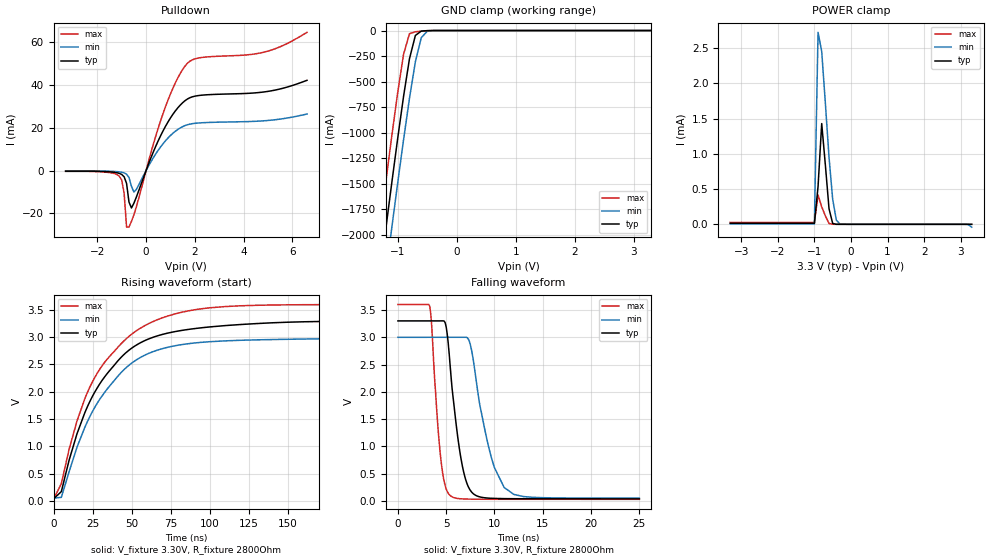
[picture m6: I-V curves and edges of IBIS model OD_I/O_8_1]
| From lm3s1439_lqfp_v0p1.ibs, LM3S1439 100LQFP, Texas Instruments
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[Model]   OD_I/O_8_1
Model_type   I/O_open_drain
Polarity   Inverting
Vinl = 1.26
Vinh = 2.04
Vmeas = 1.65
Rref = 2800
Vref = 3.3
| variable   typ   min   max
C_comp   9.739pF   9.739pF   9.739pF
[Model Spec]
Vinh+   1.91   1.78   2.04
Vinh-   1.90   1.76   2.03
Vinl+   1.40   1.27   1.54
Vinl-   1.39   1.26   1.53
| variable   typ   min   max
[Temperature Range]  25   85   -40
[Voltage Range]   3.3V   3.0V   3.6V
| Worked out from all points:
|   slope of the pulldown table from 0 to 0.495 V, typ, clamps not added: 35.8 ohm
|   GND clamp passes 1 mA (typ) near -0.48 V on its own axis
|   POWER clamp passes 1 mA (typ) near -0.73 V on its own axis
|   falling waveform, V_fixture 3.30V, R_fixture 2800Ohm: 20-80 % time 1.29ns typ, 1.99ns min, 858ps max; typ from 3.3 V to 0.038 V
|   rising waveform, V_fixture 3.30V, R_fixture 2800Ohm: 20-80 % time 34.3ns typ, 34ns min, 35.1ns max; typ from 0.038 V to 3.3 V
[Pulldown]
|  Voltage   I(typ)   I(min)   I(max)
-3.3V     -256.6uA   -145.6uA   -364.5uA
-1.1V     -1.273mA   -587.5uA   -2.567mA
-900mV    -2.885mA   -1.061mA   -10.54mA
-800mV    -5.993mA   -1.67mA    -26.39mA
-700mV    -14.71mA   -3.215mA   -26.33mA
-600mV    -17.43mA   -7.321mA   -23.73mA
-500mV    -15.26mA   -10mA      -20.66mA
700mV     18.62mA    12.61mA    26.75mA
1.2V      27.84mA    18.36mA    40.91mA
1.7V      33.44mA    21.41mA    50.13mA
4.9V      36.8mA     23.3mA     55.47mA
6.6V      42.15mA    26.42mA    64.53mA
[GND Clamp]
|  Voltage   I(typ)   I(min)   I(max)
-3.3V     -11.72A    -12.12A    -11.3A
-1.4V     -2.845A    -3.285A    -2.387A
-1.3V     -2.39A     -2.831A    -1.93A
-1.2V     -1.938A    -2.38A     -1.478A
-1.1V     -1.494A    -1.934A    -1.036A
-1V       -1.059A    -1.496A    -610.6mA
-900mV    -645mA     -1.069A    -232.9mA
-800mV    -277.1mA   -664.4mA   -31.59mA
-700mV    -48.56mA   -306.6mA   -12.09mA
-600mV    -5.558mA   -70.2mA    -6.272mA
-500mV    -1.167mA   -7.88mA    -2.167mA
3.3V      2.282nA    3.101uA    451.3pA
[POWER Clamp]
|  Voltage   I(typ)   I(min)   I(max)
-3.3V     15.18uA    8.315uA    27.48uA
-1V       14.14uA    7.74uA     25.63uA
-900mV    536uA      2.726mA    416.7uA
-800mV    1.43mA     2.454mA    247.6uA
-700mV    840.7uA    1.719mA    119.9uA
-600mV    221.2uA    951.5uA    11.58uA
-500mV    12.35uA    355.6uA    955.3nA
-400mV    305.2nA    58.59uA    44.3nA
-300mV    9.515nA    3.101uA    1.472nA
3.1V      1.302nA    -112.7nA   143.5pA
3.2V      1.207nA    -2.287uA   131.7pA
3.3V      -104.8pA   -40.34uA   119.2pA
[Ramp]
| variable   typ   min   max
dV/dt_f   1.96/1.29n   1.77/1.99n   2.14/0.86n
dV/dt_r   1.96/34.30n   1.77/33.98n   2.14/35.07n
R_load = 2800Ohm
[Falling Waveform]
V_fixture = 3.30V
V_fixture_min = 3.00V
V_fixture_max = 3.60V
R_fixture = 2800Ohm
|   Time   V(typ)   V(min)   V(max)
0s        3.3V       2.999V     3.6V
3.3ns     3.3V       2.999V     3.564V
4.4ns     3.3V       2.999V     836.8mV
5ns       3.185V     2.999V     218.4mV
5.4ns     2.495V     2.999V     100.8mV
6.6ns     707.6mV    2.999V     38.13mV
7.9ns     119.4mV    2.47V      32.01mV
9.4ns     51.42mV    986.6mV    30.54mV
11ns      42.38mV    246.7mV    30.11mV
25ns      37.9mV     50.24mV    29.43mV
[Rising Waveform]
V_fixture = 3.30V
V_fixture_min = 3.00V
V_fixture_max = 3.60V
R_fixture = 2800Ohm
|   Time   V(typ)   V(min)   V(max)
0s        38mV       50.65mV    29.45mV
5ns       171.3mV    65.99mV    317.2mV
10ns      749.5mV    538.2mV    948.3mV
15ns      1.229V     982.4mV    1.463V
26ns      1.975V     1.694V     2.24V
44ns      2.653V     2.374V     2.902V
61ns      2.969V     2.704V     3.25V
83ns      3.129V     2.868V     3.463V
110ns     3.213V     2.933V     3.562V
250ns     3.298V     2.994V     3.599V
